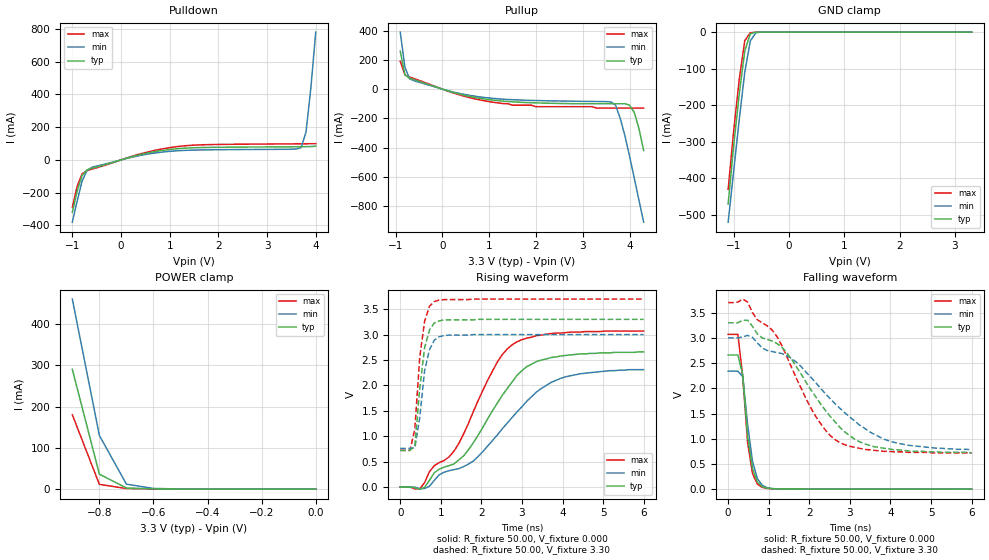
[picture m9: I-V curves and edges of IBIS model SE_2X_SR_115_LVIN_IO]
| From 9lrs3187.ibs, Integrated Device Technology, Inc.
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|   Model SE_2X_SR_115_LVIN_IO
[Model]   SE_2X_SR_115_LVIN_IO
Model_type   I/O
Polarity   Inverting
Vinl =   0.35V
Vinh =   0.7V
Vmeas =   1.50V
Cref =   5.00pF
Rref =  50.000
Vref =   1.50V
C_comp   3.40pF   2.85pF   3.95pF
[Temperature Range]   27.00   70.00   0.000
[Voltage Range]   3.30V   3.00V   3.70V
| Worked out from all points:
|   slope of the pulldown table from 0 to 0.495 V, typ, clamps not added: 12.7 ohm
|   slope of the pullup table from 0 to 0.495 V, typ, clamps not added: 11.3 ohm
|   GND clamp passes 1 mA (typ) near -0.61 V on its own axis
|   POWER clamp passes 1 mA (typ) near -0.61 V on its own axis
|   rising waveform, R_fixture 50.00, V_fixture 0.000: 20-80 % time 1.37ns typ, 1.63ns min, 1.16ns max; typ from 0 V to 2.66 V
|   rising waveform, R_fixture 50.00, V_fixture 3.30: 20-80 % time 210ps typ, 228ps min, 199ps max; typ from 0.72 V to 3.3 V
|   falling waveform, R_fixture 50.00, V_fixture 0.000: 20-80 % time 203ps typ, 224ps min, 214ps max; typ from 2.66 V to 0 V
|   falling waveform, R_fixture 50.00, V_fixture 3.30: 20-80 % time 1.38ns typ, 1.71ns min, 1.13ns max; typ from 3.3 V to 0.72 V
[Pulldown]
| voltage   I(typ)   I(min)   I(max)
|  -3.30   -4.15A   -4.00A   -4.25A
|  -3.10   -3.81A   -3.68A   -3.90A
|  -2.90   -3.47A   -3.36A   -3.55A
|  -2.70   -3.13A   -3.04A   -3.19A
|  -2.50   -2.79A   -2.72A   -2.84A
|  -2.30   -2.46A   -2.40A   -2.49A
|  -2.10   -2.12A   -2.08A   -2.14A
|  -1.90   -1.78A   -1.77A   -1.79A
|  -1.70   -1.45A   -1.45A   -1.45A
|  -1.50   -1.12A   -1.14A   -1.10A
-1V       -320mA     -380mA     -290mA
-900mV    -190mA     -250mA     -160mA
-800mV    -94.69mA   -130mA     -84.74mA
-700mV    -60.71mA   -64.73mA   -65.52mA
-600mV    -51.06mA   -45.2mA    -56.5mA
400mV     32.6mA     27.52mA    37.03mA
1.2V      69.5mA     56.57mA    82.87mA
3.5V      80.08mA    65.45mA    97.87mA
3.7V      80.56mA    75.12mA    98.32mA
3.8V      80.96mA    170mA      98.58mA
3.9V      81.72mA    440mA      98.88mA
4V        83.73mA    780mA      99.22mA
|   4.10   0.11A   1.16A   99.62mA
|   4.20   0.31A   1.55A   0.10A
|   4.30   0.66A   1.95A   0.10A
|   4.50   1.46A   2.77A   0.11A
|   4.70   2.32A   3.59A   0.58A
|   4.90   3.19A   4.43A   1.41A
|   5.10   4.07A   5.27A   2.30A
|   5.30   4.96A   6.11A   3.20A
|   5.50   5.85A   6.96A   4.12A
|   5.70   6.75A   7.81A   5.04A
|   5.90   7.64A   8.66A   5.97A
|   6.10   8.54A   9.51A   6.89A
|   6.60   10.80A   11.65A   9.23A
[Pullup]
| voltage   I(typ)   I(min)   I(max)
|  -3.30   10.68A   10.27A   10.94A
|  -3.10   9.78A   9.42A   10.01A
|  -2.90   8.88A   8.57A   9.08A
|  -2.70   7.99A   7.73A   8.16A
|  -2.50   7.09A   6.88A   7.23A
|  -2.30   6.20A   6.04A   6.30A
|  -2.10   5.31A   5.20A   5.38A
|  -1.90   4.42A   4.36A   4.46A
|  -1.70   3.54A   3.53A   3.55A
|  -1.50   2.67A   2.70A   2.64A
|  -1.00   0.59A   0.73A   0.50A
-900mV    260mA      390mA      190mA
-800mV    98.09mA    150mA      96.73mA
-700mV    74.34mA    69.92mA    82.79mA
-600mV    63.81mA    56.49mA    71.52mA
500mV     -44.25mA   -37.82mA   -51.47mA
1.5V      -86.95mA   -72.42mA   -110mA
3.5V      -100mA     -85.41mA   -130mA
3.7V      -100mA     -110mA     -130mA
3.9V      -100mA     -320mA     -130mA
4.1V      -160mA     -610mA     -130mA
4.2V      -270mA     -760mA     -130mA
4.3V      -420mA     -910mA     -130mA
|   4.50   -0.73A   -1.22A   -0.15A
|   4.70   -1.06A   -1.54A   -0.40A
|   4.90   -1.39A   -1.85A   -0.72A
|   5.10   -1.72A   -2.17A   -1.06A
|   5.30   -2.06A   -2.49A   -1.40A
|   5.50   -2.39A   -2.81A   -1.75A
|   5.70   -2.73A   -3.13A   -2.10A
|   5.90   -3.07A   -3.45A   -2.45A
|   6.10   -3.41A   -3.77A   -2.80A
|   6.60   -4.26A   -4.58A   -3.68A
[GND_clamp]
| voltage   I(typ)   I(min)   I(max)
|  -3.30   -4.15A   -4.00A   -4.25A
|  -3.20   -3.98A   -3.84A   -4.07A
|  -3.10   -3.81A   -3.68A   -3.90A
|  -3.00   -3.64A   -3.52A   -3.72A
|  -2.90   -3.47A   -3.36A   -3.55A
|  -2.80   -3.30A   -3.20A   -3.37A
|  -2.70   -3.13A   -3.04A   -3.19A
|  -2.60   -2.96A   -2.88A   -3.02A
|  -2.50   -2.79A   -2.72A   -2.84A
|  -2.40   -2.62A   -2.56A   -2.67A
|  -2.30   -2.45A   -2.40A   -2.49A
|  -2.20   -2.29A   -2.24A   -2.32A
|  -2.10   -2.12A   -2.08A   -2.14A
|  -2.00   -1.95A   -1.92A   -1.97A
|  -1.90   -1.78A   -1.76A   -1.79A
|  -1.80   -1.61A   -1.61A   -1.62A
|  -1.70   -1.45A   -1.45A   -1.45A
|  -1.60   -1.28A   -1.29A   -1.27A
|  -1.50   -1.12A   -1.14A   -1.10A
|  -1.40   -0.95A   -0.98A   -0.93A
|  -1.30   -0.79A   -0.83A   -0.76A
|  -1.20   -0.63A   -0.67A   -0.59A
-1.1V     -470mA     -520mA     -430mA
-1V       -310mA     -380mA     -270mA
-900mV    -170mA     -240mA     -130mA
-800mV    -52.1mA    -110mA     -23.59mA
-700mV    -4.69mA    -24.29mA   -1.84mA
-600mV    -430uA     -1.9mA     -210uA
-400mV    -1.76uA    -10.19uA   -470nA
3.3V      150pA      24.14uA    -330pA
[POWER_clamp]
| voltage   I(typ)   I(min)   I(max)
|  -3.30   13.34A   12.83A   13.67A
|  -3.20   12.78A   12.30A   13.09A
|  -3.10   12.22A   11.77A   12.51A
|  -3.00   11.66A   11.24A   11.93A
|  -2.90   11.10A   10.71A   11.35A
|  -2.80   10.54A   10.18A   10.77A
|  -2.70   9.98A   9.66A   10.19A
|  -2.60   9.42A   9.13A   9.61A
|  -2.50   8.86A   8.60A   9.03A
|  -2.40   8.31A   8.07A   8.46A
|  -2.30   7.75A   7.54A   7.88A
|  -2.20   7.19A   7.02A   7.30A
|  -2.10   6.64A   6.49A   6.73A
|  -2.00   6.08A   5.97A   6.15A
|  -1.90   5.53A   5.45A   5.58A
|  -1.80   4.97A   4.92A   5.00A
|  -1.70   4.42A   4.40A   4.43A
|  -1.60   3.88A   3.89A   3.86A
|  -1.50   3.33A   3.37A   3.30A
|  -1.40   2.79A   2.86A   2.74A
|  -1.30   2.25A   2.35A   2.18A
|  -1.20   1.72A   1.85A   1.63A
|  -1.10   1.21A   1.37A   1.10A
|  -1.00   0.72A   0.90A   0.60A
-900mV    290mA      460mA      180mA
-800mV    36.29mA    130mA      11.65mA
-700mV    2.83mA     12.05mA    1.52mA
-600mV    760uA      1.75mA     430uA
-500mV    190uA      510uA      90.12uA
-400mV    36.78uA    130uA      14.36uA
-300mV    5.51uA     24.14uA    1.75uA
-200mV    600nA      3.69uA     140nA
-100mV    40.72nA    380nA      6.97nA
0V        150pA      200pA      160pA
[Ramp]
| variable   typ   min   max
dV/dt_r   1.59/1.36n   1.39/1.64n   1.84/1.15n
dV/dt_f   1.55/1.38n   1.33/1.70n   1.79/1.13n
R_load = 50.00
[Rising Waveform]
R_fixture = 50.00
V_fixture = 0.000
V_fixture_min = 0.000
V_fixture_max = 0.000
| time   V(typ)   V(min)   V(max)
0s        0V         1.34uV     0V
480ps     -43.33mV   -36.21mV   -37.06mV
840ps     280mV      130mV      420mV
1.32ns    450mV      340mV      700mV
1.8ns     870mV      510mV      1.48V
2.4ns     1.66V      1.03V      2.47V
2.76ns    2.07V      1.37V      2.8V
3.12ns    2.37V      1.69V      2.93V
3.96ns    2.58V      2.14V      3.03V
6ns       2.66V      2.31V      3.07V
[Rising Waveform]
R_fixture = 50.00
V_fixture = 3.30
V_fixture_min = 3.00
V_fixture_max = 3.70
| time   V(typ)   V(min)   V(max)
0s        720mV      760mV      720mV
240ps     720mV      760mV      720mV
360ps     810mV      770mV      1.14V
480ps     1.94V      1.36V      2.55V
600ps     2.74V      2.29V      3.26V
720ps     3.09V      2.7V       3.56V
840ps     3.23V      2.89V      3.65V
960ps     3.27V      2.96V      3.68V
1.2ns     3.29V      2.99V      3.69V
6ns       3.3V       3V         3.7V
[Falling Waveform]
R_fixture = 50.00
V_fixture = 0.000
V_fixture_min = 0.000
V_fixture_max = 0.000
| time   V(typ)   V(min)   V(max)
0s        2.66V      2.34V      3.07V
240ps     2.66V      2.34V      3.07V
360ps     2.27V      2.23V      2.22V
480ps     1.05V      1.28V      920mV
600ps     410mV      550mV      310mV
720ps     140mV      210mV      100mV
840ps     48.93mV    76.66mV    35.05mV
960ps     19.96mV    29.7mV     15.02mV
1.32ns    4.41mV     4.54mV     4.01mV
6ns       49.61uV    110uV      21.14uV
[Falling Waveform]
R_fixture = 50.00
V_fixture = 3.30
V_fixture_min = 3.00
V_fixture_max = 3.70
| time   V(typ)   V(min)   V(max)
0s        3.3V       3V         3.7V
360ps     3.35V      3.02V      3.77V
720ps     3.08V      2.9V       3.36V
1.08ns    2.94V      2.73V      3.16V
1.44ns    2.71V      2.65V      2.64V
2.16ns    1.83V      2.11V      1.44V
2.76ns    1.22V      1.6V       920mV
3.24ns    940mV      1.27V      810mV
3.84ns    810mV      990mV      750mV
6ns       720mV      780mV      720mV
